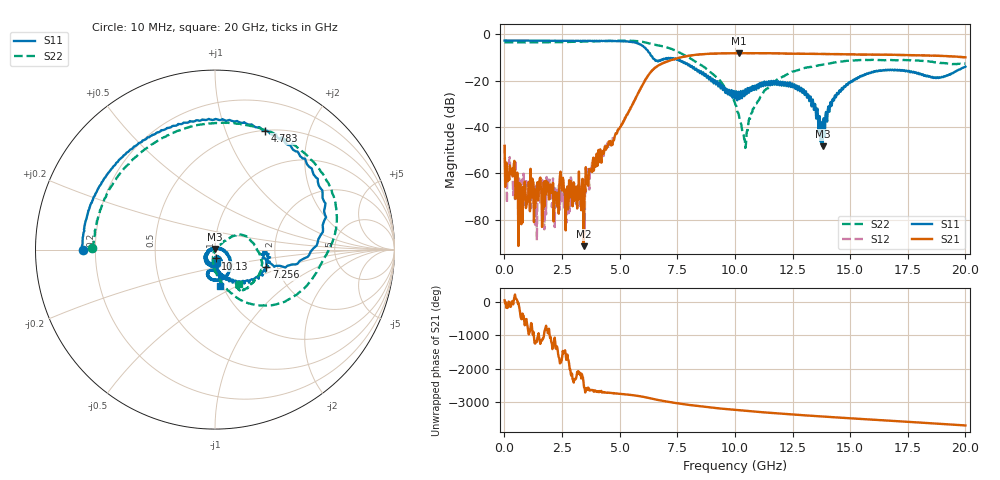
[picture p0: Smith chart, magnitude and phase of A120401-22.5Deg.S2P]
!  2-Port S-parameters saved by WinCal
! VAR MeasName=S-Parameters (CALIBRATED_DATA) read from VNA (N5244A)
! VAR MeasDate=11/21/2012 9:56:43 AM
! VAR NAME=A120401-22.5Deg
! VAR FILENAME=A120401-22.5Deg.S2P
! VAR DATE=11/21/2012 9:56:43 AM
! VAR PHYS_PORTS=1,2
# Hz S MA R 50
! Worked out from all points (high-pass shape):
!   801 points, 10 MHz to 20 GHz, reference 50 ohm
!   highest |S21| = -8.06 dB at 10.18 GHz (marker M1); lowest = -91.4 dB at 3.433 GHz (marker M2)
!   |S21| within 3 dB of the highest: 7.244 GHz to end of sweep
!   lowest |S11| = -48.4 dB at 13.8 GHz (marker M3), VSWR 1.01, Z = 49.9 + j0.357 ohm
!   |S11| at or under -10 dB: 6.435 GHz to end of sweep
!   |S22| runs from -49.0 to -2.7 dB; largest |S21 - S12| = 0.0038
!   S11 on the Smith chart (normalised r, x): 10 MHz: 0.15, -0.00; 4.783 GHz: 0.51, +1.39; 7.256 GHz: 1.75, -0.37; 10.13 GHz: 1.00, -0.10; 20 GHz: 0.97, -0.40
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1e7  0.7379 -179.9  0.003938 40.0  0.004104 96.9  0.6827 179.1
6.846625e8  0.7368 166.7  0.000604 17.7  0.0004678 -85.1  0.6751 163.5
1.159425e9  0.7352 157.6  0.0005457 80.5  0.0001774 -106.6  0.6758 152.1
2.233888e9  0.7305 135.8  0.0003481 32.5  0.0004411 123.0  0.681 125.9
2.483762e9  0.7301 130.4  0.0005529 39.8  0.0005403 58.7  0.6837 119.7
3.358325e9  0.7246 109.9  0.0004973 -0.4  0.0004218 -120.2  0.7012 97.7
3.433288e9  0.7265 108.4  2.683e-05 92.7  0.0002435 115.2  0.7015 95.7
4.782612e9  0.7189 67.0  0.006185 138.8  0.006662 139.2  0.7272 57.0
5.782112e9  0.6425 17.6  0.05153 62.2  0.05205 63.0  0.7194 21.0
6.681662e9  0.2632 -6.5  0.2134 -62.0  0.2142 -61.7  0.5795 -12.8
7.256375e9  0.3009 -18.5  0.281 -131.9  0.2816 -131.8  0.4869 -36.5
8.680662e9  0.1274 -80.3  0.377 95.9  0.3768 96.1  0.1947 -77.7
1.0005e10  0.04127 -82.6  0.3934 3.2  0.3943 3.1  0.03247 -106.0
1.012994e10  0.04948 -85.3  0.395 -4.7  0.3943 -4.6  0.0204 -104.7
1.017991e10  0.05151 -61.0  0.3952 -7.8  0.3943 -7.8  0.01739 -116.1
1.045478e10  0.06556 -71.1  0.3931 -24.4  0.3938 -24.3  0.003541 -49.4
1.127936e10  0.09651 -76.5  0.3926 -70.8  0.3933 -70.8  0.0614 43.2
1.335332e10  0.03364 179.4  0.3812 -173.3  0.381 -173.4  0.2018 16.4
1.38031e10  0.003815 110.2  0.3794 166.2  0.3786 166.1  0.2214 6.4
1.472764e10  0.07518 -22.3  0.3738 125.2  0.3747 125.1  0.2645 -12.4
1.667666e10  0.1692 -82.0  0.364 42.4  0.3647 42.2  0.2811 -39.8
2e10  0.2017 -82.6  0.3209 -100.7  0.3208 -101.0  0.2352 -55.5
